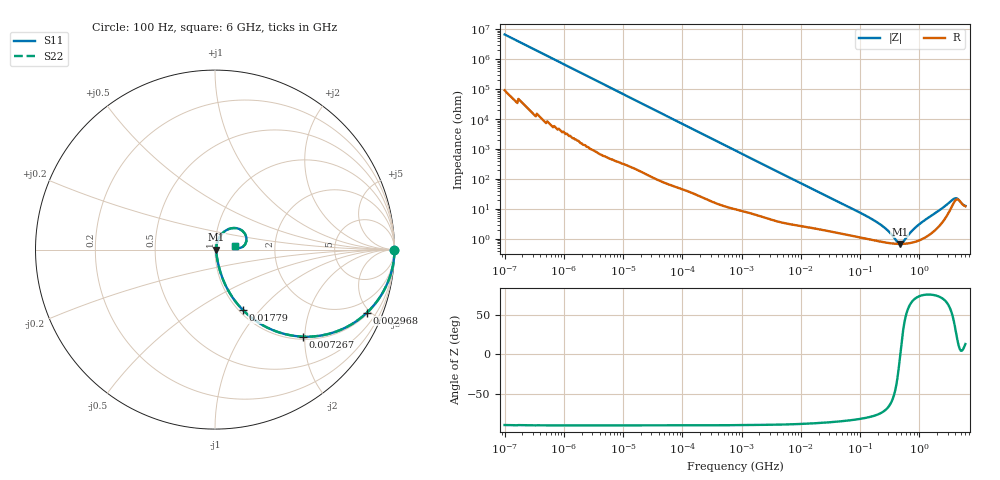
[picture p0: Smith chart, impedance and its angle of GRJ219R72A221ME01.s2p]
!Murata Part Number: GRJ219R72A221ME01
!These Parameters are Measured in Series Mode Connection
!Data Generated on Jun 19, 2026
!  o--ll--o
!Port1  Port2
!  o------o
!Operation Temp=25[degC], DC Bias Voltage=0[V]
!Freq. Start=100[Hz] Stop=6[GHz] 401[Steps]
# Hz S RI R 50
!Freq.(Hz) S11(Real) S11(Imag) S21(Real) S21(Imag) S12(Real) S12(Imag) S22(Real) S22(Imag)
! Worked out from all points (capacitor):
!   401 points, 100 Hz to 6 GHz, reference 50 ohm
!   read as one part in series: C = 234 pF near 109 Hz
!   lowest |Z| = 677 mohm at 467.5 MHz (marker M1)
!   series resonance near 477.6 MHz, so ESL is about 480 pH
!   S11 on the Smith chart (normalised r, x): 100 Hz: open; 2.968 MHz: 1.09, -4.78; 7.267 MHz: 1.06, -1.97; 17.79 MHz: 1.04, -0.81; 6 GHz: 1.25, +0.06
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100  1 -1.47e-05  2e-07 1.47e-05  2e-07 1.47e-05  1 -1.47e-05
656  1 -9.56e-05  5e-07 9.56e-05  5e-07 9.56e-05  1 -9.56e-05
2008  1 -0.000292  1.4e-06 0.000292  1.4e-06 0.000292  1 -0.000292
40335  0.9999 -0.00581  6.39e-05 0.00581  6.39e-05 0.00581  0.9999 -0.00581
774597  0.9868 -0.1088  0.0132 0.1088  0.0132 0.1088  0.9868 -0.1088
1658239  0.9446 -0.2212  0.0554 0.2212  0.0554 0.2212  0.9446 -0.2212
2967816  0.8463 -0.3514  0.1537 0.3514  0.1537 0.3514  0.8463 -0.3514
7266822  0.4917 -0.4851  0.5083 0.4851  0.5083 0.4851  0.4917 -0.4851
1.555665e7  0.1893 -0.3679  0.8107 0.3679  0.8107 0.3679  0.1893 -0.3679
1.779312e7  0.1553 -0.3364  0.8447 0.3364  0.8447 0.3364  0.1553 -0.3364
3.80911e7  0.0504 -0.1806  0.9496 0.1806  0.9496 0.1806  0.0504 -0.1806
1.334425e8  0.0126 -0.0531  0.9874 0.0531  0.9874 0.0531  0.0126 -0.0531
2.183701e8  0.00885 -0.0288  0.9912 0.0288  0.9912 0.0288  0.00885 -0.0288
3.124326e8  0.00734 -0.0149  0.9927 0.0149  0.9927 0.0149  0.00734 -0.0149
4.674818e8  0.00668 -0.000741  0.9933 0.000741  0.9933 0.000741  0.00668 -0.000741
5.346885e8  0.00673 0.00397  0.9933 -0.00397  0.9933 -0.00397  0.00673 0.00397
7.31507e8  0.0075 0.0155  0.9925 -0.0155  0.9925 -0.0155  0.0075 0.0155
1.000774e9  0.00961 0.0289  0.9904 -0.0289  0.9904 -0.0289  0.00961 0.0289
2.34314e9  0.0387 0.0878  0.9613 -0.0878  0.9613 -0.0878  0.0387 0.0878
3.505958e9  0.1193 0.1194  0.8807 -0.1194  0.8807 -0.1194  0.1193 0.1194
4.193612e9  0.1748 0.0691  0.8252 -0.0691  0.8252 -0.0691  0.1748 0.0691
6e9  0.1099 0.0224  0.8901 -0.0224  0.8901 -0.0224  0.1099 0.0224
